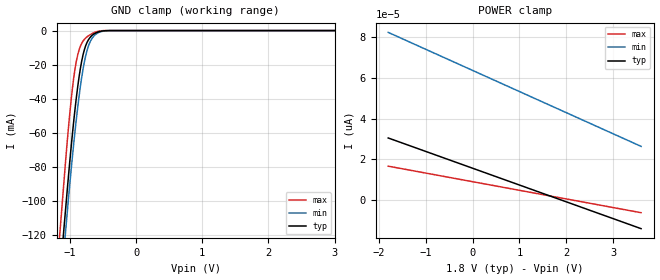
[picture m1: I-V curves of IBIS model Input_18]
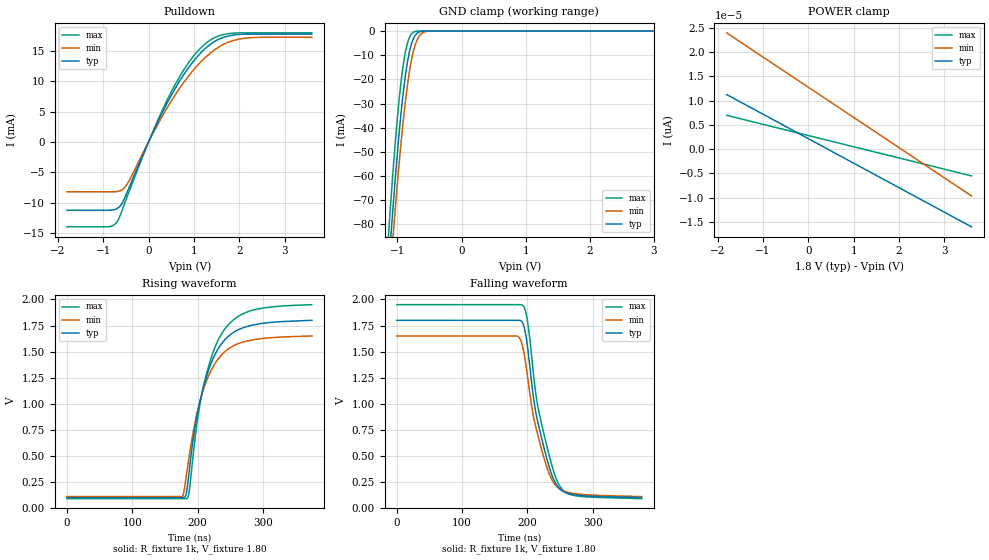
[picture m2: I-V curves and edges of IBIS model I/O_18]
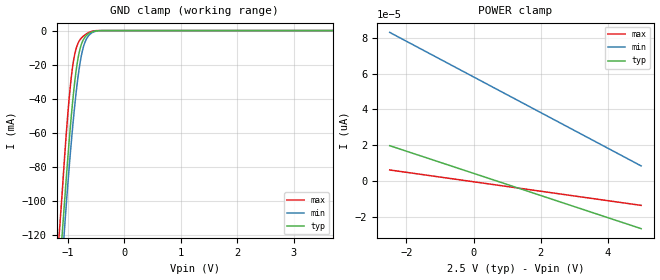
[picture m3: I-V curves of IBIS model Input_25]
|//////////////////////////////////////////////////////////////////////////////
|//////////////////////////////////////////////////////////////////////////////
|   @@@@@@@   @@@@@@@   @@@@@@@   @@@@@@@   @@@@@@@   @@@@@@   @@
|   @@@@@@@@@   @@@@@@@@@   @@@@@@@@@   @@@@@@@@@   @@@@@@@@@ @@@@@@@@  @
|   @@@   @@@ @@@   @@@ @@@   @@@   @@@ @@@   @@@@   @@@  @
|   @@   @@ @@   @@ @@@@@@@@@@@ @@@@@@@@@@@ @@   @@   @@ @@
|   @@@   @@@ @@   @@   @@@ @@@   @@   @@   @@ @@
|   @@@@@@@@@  @@   @@  @@@@@@@@@   @@@@@@@@@  @@   @@   @@ @@
|   @@@@@@@   @@   @@   @@@@@@@   @@@@@@@   @@   @@   @@ @@
|   IBIS Model of N24S64
|   64 Kb I2C CMOS Serial EEPROM with Software Write Protect
|   and Programmable Device Address
|   WLCSP-4  Package Type, CASE 567VX, C4 SUFFIX
|   The model is covering the following Vccs:
|   1.8V, 2.5V, 3.3V, 5.0V
|//////////////////////////////////////////////////////////////////////////////
|//////////////////////////////////////////////////////////////////////////////
[IBIS Ver]   3.2
|   7.1 compatible
|//////////////////////////////////////////////////////////////////////////////
[Comment Char] |_char
|//////////////////////////////////////////////////////////////////////////////
[File Name]   n24s64_gc_r0.ibs
|//////////////////////////////////////////////////////////////////////////////
[File Rev]   0.0
|   0.0 - Jun 27, 2023 - File created
|//////////////////////////////////////////////////////////////////////////////
[Date]   June 27, 2023
|//////////////////////////////////////////////////////////////////////////////
[Source]   From lab measurements at onsemi
|//////////////////////////////////////////////////////////////////////////////
[Notes]
   - The currents greater than +/- 100 mA are extrapolated
|//////////////////////////////////////////////////////////////////////////////
[Disclaimer]
   - onsemi Corporation hereby grants
   the user of this IBIS model a license to use this IBIS
   model under the following terms. This license in nonexclusive
   and nontransferable. Before using this IBIS model.
   After reading the terms and conditions of this license,
   the user either must accept these terms,
   or the IBIS model should be returned to onsemi within 30 days.
   - The user is hereby granted a license to use the IBIS model.
   This shall not be construed as a right to sell,
   or otherwise profit either by leasing or renting this software.
   - The user may modify the IBIS model to suit his specific
   applications but rights to derivative works and such
   modifications shall belong to onsemi.
   - This IBIS model is provided on an "as is" basis.
   onsemi makes absolutely no warranty with respect
   to the information contained herein.
   By use of this IBIS model, the user assumes full risk as to the
   quality and suitablility of the model to his particular use,
   and by using this model assumes the entire risk.
   Under all circumstances the user shall not hold
   onsemi liable in any way for the results obtained.
   onsemi reserves the right to make to improve
   the model for reliability, function, or design.
   onsemi does not convey any license under patent
   rights or any other intellectual property rights,
   including those of third parties.
   - onsemi is not obligated to provide maintenance
   or support for the licensed IBIS model.
   - Cont onsemi at ATTN:LOGIC APPLICATIONS/IBIS MODEL.
   5005 E. McDowell Road, Phoenix AZ 85008
|//////////////////////////////////////////////////////////////////////////////
[Copyright]   (c) 2023 onsemi Corp.
|//////////////////////////////////////////////////////////////////////////////
|//////////////////////////////////////////////////////////////////////////////
[Component]   N24S64C4DYT3G
|//////////////////////////////////////////////////////////////////////////////
[Manufacturer]  onsemi
|   Data Sheet: N24S64/D, Rev. 1,  Nov, 2018
|//////////////////////////////////////////////////////////////////////////////
[Package]
|  WLCSP-4
| CASE 567VX
| C4 SUFFIX
| variable   typ   min   max
R_pkg   0.0013   0.0013   0.0013
L_pkg   0.0212nH   0.0212nH   0.0212nH
C_pkg   0.0461pF   0.0461pF   0.0461pF
|//////////////////////////////////////////////////////////////////////////////
[Pin]   signal_name   model_name   R_pin   L_pin   C_pin
1A   VCC   POWER   0.0013   0.0212nH   0.0461pF
1B   SDA   I/O   0.0013   0.0212nH   0.0461pF
2A   SCL   Input   0.0013   0.0212nH   0.0461pF
2B   GND   GND   0.0013   0.0212nH   0.0461pF
|//////////////////////////////////////////////////////////////////////////////
|//////////////////////////////////////////////////////////////////////////////
[Model Selector]   Input
Input_18   Vcc = 1.80
Input_25   Vcc = 2.50
Input_33   Vcc = 3.30
Input_50   Vcc = 5.00
|//////////////////////////////////////////////////////////////////////////////
[Model Selector]   I/O
I/O_18   Vcc = 1.80
I/O_25   Vcc = 2.50
I/O_33   Vcc = 3.30
I/O_50   Vcc = 5.00
| Models and submodels in the file (8): Input_18 (Input), I/O_18 (I/O_open_drain), Input_25 (Input), I/O_25 (I/O_open_drain), Input_33 (Input), I/O_33 (I/O_open_drain), Input_50 (Input), I/O_50 (I/O_open_drain)
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|//////////////////////////////////////////////////////////////////////////////
|//////////////////////////////////////////////////////////////////////////////
[Model]  Input_18
Model_type Input
Vinh =  1.35
Vinl =  0.45
|  variable   typ   min   max
C_comp   6pF   6pF   6pF
|//////////////////////////////////////////////////////////////////////////////
[Temperature Range]   25   85   -40
|//////////////////////////////////////////////////////////////////////////////
[Voltage Range]   1.80V   1.65V   1.95V
|//////////////////////////////////////////////////////////////////////////////
[POWER Clamp Reference] 1.80V   1.65V   1.95V
|//////////////////////////////////////////////////////////////////////////////
[GND Clamp Reference]   0V   0V   0V
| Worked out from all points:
|   GND clamp passes 1 mA (typ) near -0.58 V on its own axis
|//////////////////////////////////////////////////////////////////////////////
[GND Clamp]
|   Voltage   I(typ)   I(min)   I(max)
-1.8V     -436.9mA   -443.7mA   -430.8mA
-1.17V    -152.8mA   -164.9mA   -128.4mA
-1.14V    -139.3mA   -151.6mA   -114mA
-1.1V     -121.3mA   -133.9mA   -94.5mA
-1.06V    -103.2mA   -116.2mA   -74.98mA
-980mV    -68.49mA   -81.82mA   -40.94mA
-900mV    -39.05mA   -51.6mA    -17.78mA
-800mV    -14.24mA   -22.69mA   -6.192mA
-740mV    -6.994mA   -11.75mA   -3.68mA
-680mV    -3.429mA   -5.607mA   -2.134mA
-420mV    -21.74uA   -54.38uA   -1.786uA
3.6V      30.48pA    83.95pA    15.98pA
|//////////////////////////////////////////////////////////////////////////////
[POWER Clamp]
|   Voltage   I(typ)   I(min)   I(max)
-1.8V     30.48pA    82.4pA     16.62pA
0V        15.62pA    63.71pA    8.991pA
1.8V      753.5fA    45.03pA    1.365pA
3.6V      -14.11pA   26.35pA    -6.261pA
|//////////////////////////////////////////////////////////////////////////////
|//////////////////////////////////////////////////////////////////////////////
[Model] I/O_18
Model_type I/O_open_drain
Vinh =  1.35
Vinl =  0.45
Vmeas = 0.90
Vref = 1.80
Rref = 1000
Cref = 100pF
|  variable   typ   min   max
C_comp   8.00pF   8.00pF   8.00pF
|//////////////////////////////////////////////////////////////////////////////
[Temperature Range]   25   85   -40
|//////////////////////////////////////////////////////////////////////////////
[Voltage Range]   1.80V   1.65V   1.95V
|//////////////////////////////////////////////////////////////////////////////
[Pulldown Reference]   0V   0V   0V
|//////////////////////////////////////////////////////////////////////////////
[POWER Clamp Reference] 1.80V   1.65V   1.95V
|////////////////////////////////////////////////////////////////////////
[GND Clamp Reference]   0V   0V   0V
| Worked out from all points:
|   slope of the pulldown table from 0 to 0.27 V, typ, clamps not added: 61.9 ohm
|   GND clamp passes 1 mA (typ) near -0.70 V on its own axis
|   falling waveform, R_fixture 1k, V_fixture 1.80: 20-80 % time 29.4ns typ, 30ns min, 30.7ns max; typ from 1.8 V to 0.1 V
|   rising waveform, R_fixture 1k, V_fixture 1.80: 20-80 % time 36.9ns typ, 37.3ns min, 36.7ns max; typ from 0.1 V to 1.8 V
|//////////////////////////////////////////////////////////////////////////////
[Pulldown]
|   Voltage   I(typ)   I(min)   I(max)
-1.8V     -11.27mA   -8.232mA   -14.01mA
-870mV    -11.26mA   -8.232mA   -13.98mA
-690mV    -10.98mA   -8.187mA   -13.12mA
-570mV    -9.927mA   -7.797mA   -10.96mA
-440mV    -7.702mA   -6.549mA   -8.372mA
80mV      1.341mA    1.176mA    1.443mA
440mV     6.857mA    6.004mA    7.378mA
880mV     12.24mA    10.86mA    13.05mA
1.28V     15.61mA    14.12mA    16.37mA
1.6V      17.1mA     15.88mA    17.61mA
2V        17.72mA    16.96mA    17.98mA
3.6V      17.78mA    17.25mA    17.99mA
|//////////////////////////////////////////////////////////////////////////////
[GND Clamp]
|   Voltage   I(typ)   I(min)   I(max)
-1.8V     -346.9mA   -351.1mA   -342.5mA
-1.14V    -98.98mA   -110.2mA   -84.68mA
-1.1V     -84.09mA   -95.8mA    -69.26mA
-1.06V    -69.95mA   -82.21mA   -54.95mA
-980mV    -44.19mA   -56.75mA   -30.11mA
-920mV    -28.03mA   -39.89mA   -16.05mA
-880mV    -19.28mA   -30.1mA    -9.26mA
-820mV    -9.449mA   -18mA      -3.126mA
-740mV    -2.57mA    -7.225mA   -335uA
-640mV    -201uA     -1.439mA   -5.478uA
-520mV    -2.591uA   -68.79uA   -28.24nA
3.6V      11.26pA    24.9pA     6.629pA
|//////////////////////////////////////////////////////////////////////////////
[POWER Clamp]
|   Voltage   I(typ)   I(min)   I(max)
-1.8V     11.26pA    23.97pA    6.975pA
0V        2.172pA    12.77pA    2.817pA
1.8V      -6.911pA   1.574pA    -1.341pA
3.6V      -15.99pA   -9.625pA   -5.5pA
|//////////////////////////////////////////////////////////////////////////////
|//////////////////////////////////////////////////////////////////////////////
[Ramp]
|  variable   typ   min   max
dV/dt_r   1.020E+00/3.750E-08  9.240E-01/3.750E-08  1.116E+00/3.600E-08
dV/dt_f   1.020E+00/3.000E-08  9.240E-01/3.000E-08  1.116E+00/3.000E-08
R_load = 1k
|//////////////////////////////////////////////////////////////////////////////
|//////////////////////////////////////////////////////////////////////////////
[Falling Waveform]
R_fixture = 1k
V_fixture = 1.80
V_fixture_min = 1.65
V_fixture_max = 1.95
C_fixture = 0p
|   time   V(typ)   V(min)   V(max)
0s        1.8V       1.65V      1.95V
183ns     1.8V       1.65V      1.95V
193.5ns   1.764V     1.526V     1.939V
201ns     1.504V     1.221V     1.755V
208.5ns   1.095V     904.6mV    1.33V
214.5ns   863.1mV    734.6mV    1.026V
232.5ns   412.7mV    344.1mV    525.4mV
249ns     187.2mV    184.6mV    216.6mV
274.5ns   125mV      137.1mV    117.4mV
375ns     100mV      110mV      90mV
|//////////////////////////////////////////////////////////////////////////////
[Rising Waveform]
R_fixture = 1k
V_fixture = 1.80
V_fixture_min = 1.65
V_fixture_max = 1.95
C_fixture = 0p
|   time   V(typ)   V(min)   V(max)
0s        100mV      110mV      90mV
175.5ns   100mV      110mV      90mV
184.5ns   213.1mV    386.3mV    95.67mV
187.5ns   372.2mV    510.4mV    176.5mV
196.5ns   797.7mV    833.1mV    689.5mV
208.5ns   1.145V     1.13V      1.157V
223.5ns   1.431V     1.353V     1.491V
238.5ns   1.59V      1.48V      1.688V
282ns     1.751V     1.61V      1.893V
375ns     1.8V       1.65V      1.95V
|//////////////////////////////////////////////////////////////////////////////
|//////////////////////////////////////////////////////////////////////////////
[Model]  Input_25
Model_type Input
Vinh =  1.75
Vinl =  0.75
|  variable   typ   min   max
C_comp   6pF   6pF   6pF
|//////////////////////////////////////////////////////////////////////////////
[Temperature Range]   25   85   -40
|//////////////////////////////////////////////////////////////////////////////
[Voltage Range]   2.50V   2.30V   2.70V
|//////////////////////////////////////////////////////////////////////////////
[POWER Clamp Reference] 2.50V   2.30V   2.70V
|//////////////////////////////////////////////////////////////////////////////
[GND Clamp Reference]   0V   0V   0V
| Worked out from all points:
|   GND clamp passes 1 mA (typ) near -0.59 V on its own axis
|//////////////////////////////////////////////////////////////////////////////
[GND Clamp]
|   Voltage   I(typ)   I(min)   I(max)
-2.5V     -758.6mA   -779.6mA   -739.3mA
-1.17V    -151.7mA   -167.8mA   -127.5mA
-1.14V    -138mA     -154mA     -113.7mA
-1.1V     -119.7mA   -135.6mA   -95.32mA
-1.06V    -101.5mA   -117.2mA   -75.66mA
-1V       -74.76mA   -90.26mA   -49.05mA
-940mV    -50.81mA   -66.17mA   -27.82mA
-900mV    -37mA      -51.59mA   -17.9mA
-840mV    -20.6mA    -32.69mA   -9.228mA
-740mV    -6.417mA   -11.65mA   -3.684mA
-620mV    -1.543mA   -2.556mA   -1.02mA
5V        19.69pA    85.03pA    5.573pA
|//////////////////////////////////////////////////////////////////////////////
[POWER Clamp]
|   Voltage   I(typ)   I(min)   I(max)
-2.5V     19.69pA    83.04pA    6.101pA
0V        4.218pA    58.15pA    -498.6fA
2.5V      -11.25pA   33.26pA    -7.098pA
5V        -26.72pA   8.364pA    -13.7pA
